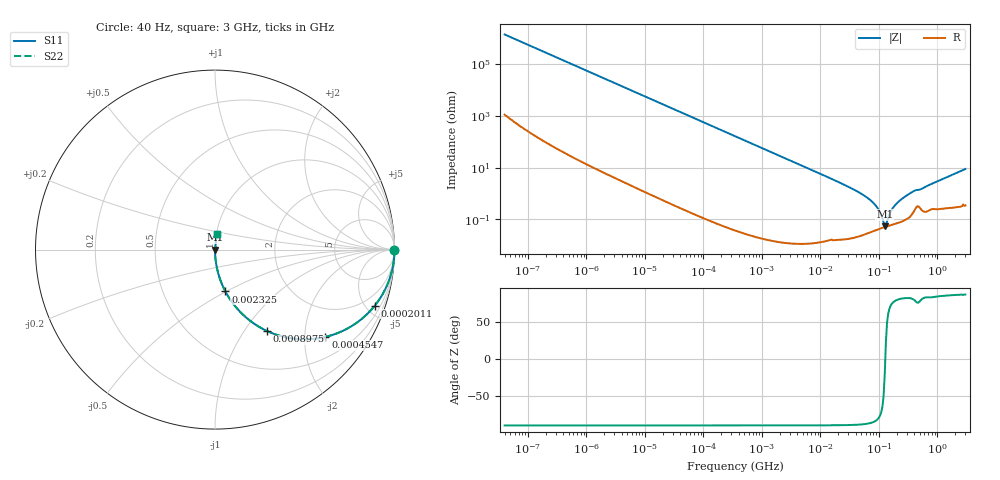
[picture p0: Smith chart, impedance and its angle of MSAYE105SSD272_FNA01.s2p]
! MSAYE105SSD272_FNA01  S-PARAMETER MODEL  ( General Type )
! Model Generated by TAIYO YUDEN Corporation (http://www.ty-top.com)
! Version 2.0
! TAIYO YUDEN Control No. 040624
! Copyright(c) 2004 TAIYO YUDEN CO.,LTD. All Rights Reserved.
! Product Description (link to TY-COMPAS)
! https://ds.yuden.co.jp/TYCOMPAS/or/detail?pn=MSAYE105SSD272KFNA01&u=M
! Products Name : Multilayer Ceramic Capacitors
! Characteristics :
!  Capacitance : 2700 pF , Rated Voltage : 16V
!  Case Size : 1.0 x 0.5 / 0.039 x 0.02 [mm/inch] , Thickness : 0.5 / 0.02 [mm/inch]
!  (Conditions: Temperature = 25 degC , DC Bias Current/Voltage = 0A / 0V)
! External Node Assignments :
!  1  o---| |---o  2
! GND o---------o GND
! Frequency Range : 40Hz  -  3GHz  [ 401 STEP ]
# MHz S RI R 50
! Freq[MHz].  S11 Real  S11 Imag  S21 Real  S21 Imag  S12 Real  S12 Imag  S22 Real  S22 Imag
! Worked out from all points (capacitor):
!   401 points, 40 Hz to 3 GHz, reference 50 ohm
!   read as one part in series: C = 2.77 nF near 44 Hz
!   lowest |Z| = 52.8 mohm at 125.6 MHz (marker M1)
!   series resonance near 128.2 MHz, so ESL is about 560 pH
!   S11 on the Smith chart (normalised r, x): 40 Hz: open; 201.1 kHz: 1.00, -5.72; 454.7 kHz: 1.00, -2.53; 897.5 kHz: 1.00, -1.28; 2.325 MHz: 1.00, -0.49; 3 GHz: 1.01, +0.18
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4e-05  1 -6.96e-05  5.9e-08 6.96e-05  5.9e-08 6.96e-05  1 -6.96e-05
6.3e-05  1 -0.00011  7.4e-08 0.00011  7.4e-08 0.00011  1 -0.00011
0.000834  1 -0.00145  2.45e-06 0.00145  2.45e-06 0.00145  1 -0.00145
0.017386  0.9991 -0.0302  0.00092 0.0302  0.00092 0.0302  0.9991 -0.0302
0.067738  0.9863 -0.1162  0.0137 0.1162  0.0137 0.1162  0.9863 -0.1162
0.201066  0.891 -0.3116  0.109 0.3116  0.109 0.3116  0.891 -0.3116
0.362475  0.7155 -0.4511  0.2845 0.4511  0.2845 0.4511  0.7155 -0.4511
0.454691  0.6151 -0.4864  0.3849 0.4864  0.3849 0.4864  0.6151 -0.4864
0.897494  0.2909 -0.4541  0.7091 0.4541  0.7091 0.4541  0.2909 -0.4541
2.325263  0.0577 -0.2329  0.9423 0.2329  0.9423 0.2329  0.0577 -0.2329
7.222098  0.00637 -0.0788  0.9936 0.0788  0.9936 0.0788  0.00637 -0.0788
30.80834  0.00048 -0.0175  0.9995 0.0175  0.9995 0.0175  0.00048 -0.0175
63.63129  0.000326 -0.0067  0.9997 0.0067  0.9997 0.0067  0.000326 -0.0067
91.44753  0.000394 -0.00302  0.9996 0.00302  0.9996 0.00302  0.000394 -0.00302
120.0322  0.000479 -0.000564  0.9995 0.000564  0.9995 0.000564  0.000479 -0.000564
125.5988  0.000495 -0.000182  0.9995 0.000182  0.9995 0.000182  0.000495 -0.000182
137.5184  0.000529 0.000629  0.9995 -0.000629  0.9995 -0.000629  0.000529 0.000629
150.5692  0.000565 0.00141  0.9994 -0.00141  0.9994 -0.00141  0.000565 0.00141
172.504  0.000623 0.00262  0.9994 -0.00262  0.9994 -0.00262  0.000623 0.00262
206.7996  0.000717 0.00429  0.9993 -0.00429  0.9993 -0.00429  0.000717 0.00429
356.2883  0.00152 0.0106  0.9985 -0.0106  0.9985 -0.0106  0.00152 0.0106
3000  0.011 0.0868  0.989 -0.0868  0.989 -0.0868  0.011 0.0868
